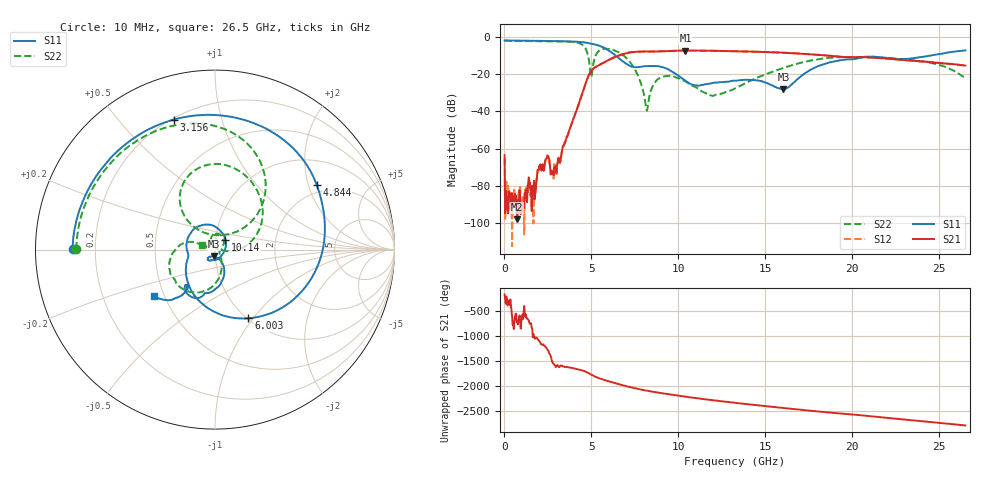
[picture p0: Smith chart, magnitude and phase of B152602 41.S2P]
!  2-Port S-parameters saved by WinCal
! VAR MeasName=S-Parameters (CALIBRATED_DATA) read from VNA (N5242A)
! VAR MeasDate=2016-1-5 16:32:08
! VAR NAME=B152602 41
! VAR FILENAME=B152602 41.S2P
! VAR DATE=2016-1-5 16:32:08
! VAR PHYS_PORTS=1,2
# Hz S DB R 50
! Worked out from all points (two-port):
!   801 points, 10 MHz to 26.5 GHz, reference 50 ohm
!   highest |S21| = -7.40 dB at 10.41 GHz (marker M1); lowest = -97.8 dB at 738.5 MHz (marker M2)
!   |S21| within 3 dB of the highest: 6.478 GHz to 18.91 GHz (12.43 GHz wide, 97.9 % of centre)
!   lowest |S11| = -28.3 dB at 16.04 GHz (marker M3), VSWR 1.08, Z = 49.3 - j3.78 ohm
!   |S11| at or under -10 dB: 6.377 GHz to 24.54 GHz (18.16 GHz wide, 118 % of centre)
!   |S22| runs from -39.6 to -2.2 dB; largest |S21 - S12| = 0.0027
!   S11 on the Smith chart (normalised r, x): 10 MHz: 0.12, +0.00; 3.156 GHz: 0.21, +0.71; 4.844 GHz: 1.72, +2.27; 6.003 GHz: 1.01, -0.95; 10.14 GHz: 1.12, +0.13; 26.5 GHz: 0.44, -0.28
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1e7  -2.01 179.7  -63.45 -171.9  -65.14 -93.3  -2.24 179.8
1.755625e8  -2.02 176.4  -92.66 -29.8  -89.57 69.9  -2.24 177.3
7.38475e8  -2.08 164.8  -97.80 5.4  -85.31 -31.0  -2.27 168.6
1.665625e9  -2.19 145.4  -84.22 122.7  -100.03 -90.4  -2.36 153.9
2.427212e9  -2.28 127.7  -65.11 -162.6  -64.62 -160.5  -2.44 140.5
3.155688e9  -2.38 107.5  -67.19 177.0  -67.39 -180.0  -2.54 125.2
4.447075e9  -2.88 55.8  -31.20 117.2  -31.19 117.2  -4.11 74.2
4.844425e9  -3.46 32.5  -20.68 57.3  -20.68 57.5  -11.88 37.5
5.0431e9  -3.85 19.7  -17.69 18.4  -17.70 18.6  -19.06 122.3
5.274888e9  -4.34 2.8  -16.04 -20.3  -16.04 -20.2  -9.40 125.5
6.003362e9  -7.42 -64.1  -12.39 -105.4  -12.39 -105.4  -6.58 78.7
7.327862e9  -16.07 -162.9  -8.26 131.4  -8.27 131.4  -14.97 7.9
8.155675e9  -15.76 166.1  -7.97 70.5  -7.95 70.4  -38.72 36.8
8.851038e9  -15.82 129.9  -7.90 29.1  -7.90 29.0  -22.56 104.7
1.014242e10  -21.85 44.0  -7.43 -38.5  -7.43 -38.5  -22.75 50.2
1.040732e10  -23.68 22.2  -7.40 -51.7  -7.41 -51.6  -23.97 38.4
1.189739e10  -24.96 -84.6  -7.56 -118.7  -7.53 -118.8  -31.50 -20.8
1.3255e10  -23.53 -113.3  -7.78 -173.5  -7.77 -173.6  -27.66 -48.7
1.603645e10  -28.26 -98.3  -8.60 83.0  -8.57 83.1  -16.79 -78.8
1.769208e10  -17.26 -67.8  -9.47 25.1  -9.45 25.3  -12.62 -102.8
2.209604e10  -11.43 -129.0  -11.84 -117.9  -11.78 -118.2  -11.50 -162.8
2.65e10  -7.35 -142.7  -15.46 94.3  -15.45 94.0  -22.32 162.3
